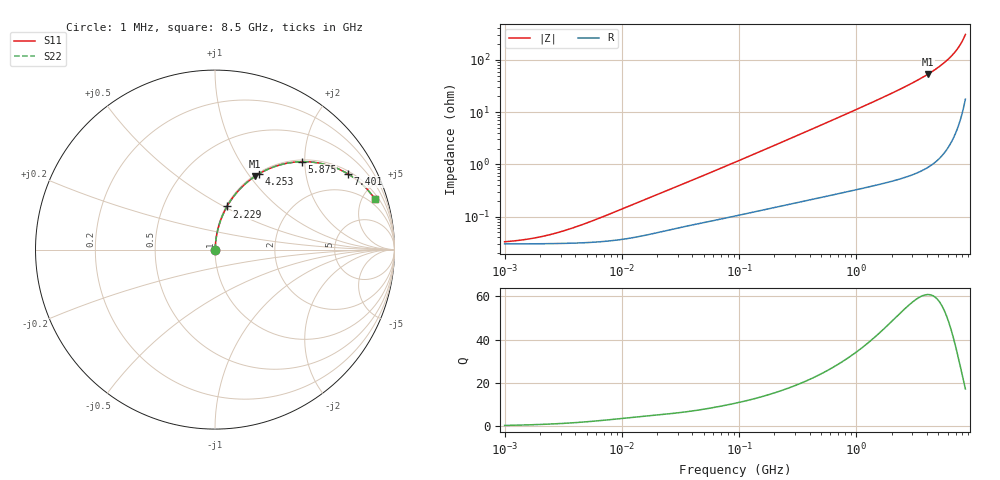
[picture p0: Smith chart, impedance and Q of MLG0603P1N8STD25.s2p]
! S-Parameter Data Generated by TDK Corporation
! Copyright(C) 2025 TDK Corporation.
! All Rights Reserved.
! TDK P/N: MLG0603P1N8STD25 (SMD / SMT Inductor (Coil))
! Property: L=1.8nH at 500MHz
! Size(LxWxT): 0.6x0.3x0.3mm
! Model Type: s2p (Touchstone File Format Version 1.0)
! Frequency: DC=Yes Start=1MHz Stop=8500MHz 198points Log-sweep
! Model Generated on Feb. 6, 2025
! Terms and conditions regarding TDK Simulation Models:
! 1)This simulation model is being provided solely for informational
!  purposes. Please refer to the specifications of the products in
!  terms of detailed characteristics of such products.
! 2)In no event shall TDK Corporation of any of its subsidiaries be
!  liable for any loss or damage arising, directly or indirectly,
!  from any information contained in this simulation model, including,
!  but not limited to loss or damages arising from any inaccuracies,
!  omissions or errors in connection with such information.
! 3)Any and all copyrights on this simulation model are owned by
!  TDK Corporation.  Duplication or redistribution of this simulation
!  model without prior written permission from TDK Corporation
!  is prohibited.
! 4)This simulation model is subject to any modification or change
!  without any prior notice.
! 5)Neither TDK Corporation nor any of its subsidiaries shall make any
!  warranty, express or implied, including but not limited to the
!  correctness, implied warranties of merchantability and fitness for
!  a particular purpose with respect to this simulation models.
! 6)The use of this simulation model shall be deemed to have consented
!  to the terms and conditions hereof.
! Port Assignments:
!  1 ---@@@--- 2
! Applicable Conditions:
!  Temperature = 25 degC
!  DC Bias Current = 0 A
!  Small Signal Operation
# Hz S MA R 50
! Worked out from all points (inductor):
!   197 points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, 1 MHz to 8.5 GHz, reference 50 ohm
!   read as one part in series: L = 2.15 nH near 7.623 MHz
!   highest Q = 60.8 at 4.061 GHz (marker M1), where L = 2.08 nH
!   S11 on the Smith chart (normalised r, x): 1 MHz: 1.00, +0.00; 2.229 GHz: 1.01, +0.52; 4.253 GHz: 1.02, +1.13; 5.875 GHz: 1.04, +1.93; 7.401 GHz: 1.11, +3.44; 8.5 GHz: 1.35, +6.13
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1000000  0.0003306 24.6  0.9997 -0.0  0.9997 -0.0  0.0003306 24.6
1446720  0.0003612 33.4  0.9997 -0.0  0.9997 -0.0  0.0003612 33.4
2092998  0.000418 43.5  0.9997 -0.0  0.9997 -0.0  0.000418 43.5
3027982  0.0005167 53.5  0.9997 -0.0  0.9997 -0.0  0.0005167 53.5
4587603  0.0007031 63.3  0.9997 -0.0  0.9997 -0.0  0.0007031 63.3
7622799  0.001091 71.7  0.9997 -0.1  0.9997 -0.1  0.001091 71.7
2.10461e7  0.002781 79.4  0.9995 -0.2  0.9995 -0.2  0.002781 79.4
9.219544e7  0.011 84.0  0.9989 -0.6  0.9989 -0.6  0.011 84.0
4.229561e8  0.04787 84.7  0.9967 -2.7  0.9967 -2.7  0.04787 84.7
9.708683e8  0.1084 82.1  0.9909 -6.2  0.9909 -6.2  0.1084 82.1
1.404574e9  0.1564 79.6  0.9839 -9.0  0.9839 -9.0  0.1564 79.6
1.940355e9  0.2165 76.3  0.9718 -12.5  0.9718 -12.5  0.2165 76.3
2.228565e9  0.2493 74.4  0.9636 -14.4  0.9636 -14.4  0.2493 74.4
3.07866e9  0.3479 68.7  0.9315 -20.4  0.9315 -20.4  0.3479 68.7
4.061159e9  0.4661 61.3  0.8771 -27.8  0.8771 -27.8  0.4661 61.3
4.253027e9  0.4896 59.7  0.8639 -29.3  0.8639 -29.3  0.4896 59.7
5.115526e9  0.5961 52.4  0.7926 -36.6  0.7926 -36.6  0.5961 52.4
5.87536e9  0.6886 45.4  0.7118 -43.5  0.7118 -43.5  0.6886 45.4
6.748056e9  0.7879 36.6  0.5966 -52.0  0.5966 -52.0  0.7879 36.6
7.400733e9  0.853 29.7  0.4956 -58.5  0.4956 -58.5  0.853 29.7
8.116539e9  0.911 21.9  0.3733 -65.5  0.3733 -65.5  0.911 21.9
8.5e9  0.9351 17.7  0.3045 -69.0  0.3045 -69.0  0.9351 17.7
